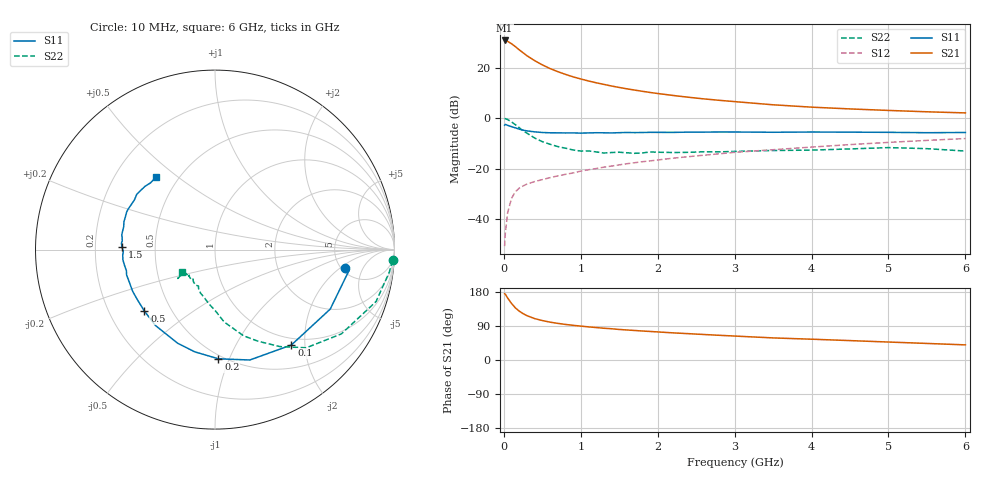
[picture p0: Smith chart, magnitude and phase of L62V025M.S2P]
!  INFINEON TECHNOLOGIES Small Signal Semiconductors
! BFR380L3 , Si-NPN RF-Transistor in TSLP-3-1
!  Vce=2 V,  Ic=25 mA
! Common Emitter S-Parameters:  07. March 2005
#  GHz  S  MA  R  50
! f  S11  S21  S12  S22
! GHz  Mag  Ang  Mag  Ang  Mag  Ang  Mag  Ang
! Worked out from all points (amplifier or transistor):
!   36 points, 10 MHz to 6 GHz, reference 50 ohm
!   highest |S21| = 30.9 dB at 10 MHz (marker M1)
!   |S21| within 3 dB of that: start of sweep to 171.7 MHz
!   unconditionally stable (mu >= 1): 1.857 GHz to 4.871 GHz
!   at 250 MHz: K = 0.39, MSG = 26.4 dB, |S12| = -26.9 dB
!   at 1.4 GHz: K = 0.96, MSG = 15.9 dB, |S12| = -19.0 dB
!   at 6 GHz: K = 0.98, MSG = 5.1 dB, |S12| = -8.0 dB
!   S11 on the Smith chart (normalised r, x): 10 MHz: 5.37, -2.30; 100 MHz: 0.88, -1.74; 200 MHz: 0.47, -0.91; 500 MHz: 0.35, -0.33; 1.5 GHz: 0.32, +0.01; 6 GHz: 0.38, +0.42
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0.01  0.7291 -7.9  34.96 174.8  0.0029 73.5  0.9912 -3.5
0.02  0.7571 -8.5  34.9 173.4  0.0054 85.2  0.9791 -7.4
0.05  0.7226 -27.3  33.5 163.3  0.0135 79.8  0.9427 -17.9
0.1  0.6809 -51.3  30.09 149.2  0.0258 68.0  0.8464 -33.7
0.15  0.6449 -72.5  26.36 137.5  0.0349 60.1  0.7468 -47.1
0.2  0.6087 -88.2  22.79 128.9  0.041 57.2  0.6504 -56.2
0.25  0.5807 -101.2  19.92 122.4  0.0453 53.3  0.5634 -64.9
0.3  0.5616 -111.8  17.43 117.0  0.0495 51.7  0.5066 -71.6
0.4  0.5376 -128.0  13.9 109.3  0.0554 50.8  0.4062 -82.8
0.5  0.5217 -138.9  11.47 104.1  0.0607 51.8  0.3436 -89.3
0.6  0.5148 -147.2  9.687 99.9  0.0662 52.5  0.305 -96.2
0.7  0.5142 -153.2  8.423 96.7  0.0719 54.3  0.2745 -102.5
0.8  0.5107 -159.1  7.436 93.9  0.0771 55.7  0.2551 -108.5
0.9  0.5124 -164.0  6.632 91.5  0.0822 56.6  0.235 -113.0
1.1  0.5122 -170.5  5.494 87.4  0.0952 58.8  0.2252 -119.0
1.5  0.5176 178.6  4.086 80.6  0.1189 61.3  0.2118 -129.4
1.8  0.5218 172.6  3.429 76.5  0.1374 62.3  0.2049 -134.9
2.2  0.5241 166.1  2.834 71.6  0.1615 62.8  0.209 -137.9
3.5  0.5275 148.4  1.85 58.3  0.2378 61.7  0.2292 -143.2
4.5  0.5299 142.0  1.532 51.2  0.3003 60.5  0.2462 -142.8
5.5  0.5169 133.9  1.344 43.7  0.3639 56.9  0.2494 -142.7
6  0.5221 128.8  1.277 39.9  0.396 54.8  0.2235 -145.4
